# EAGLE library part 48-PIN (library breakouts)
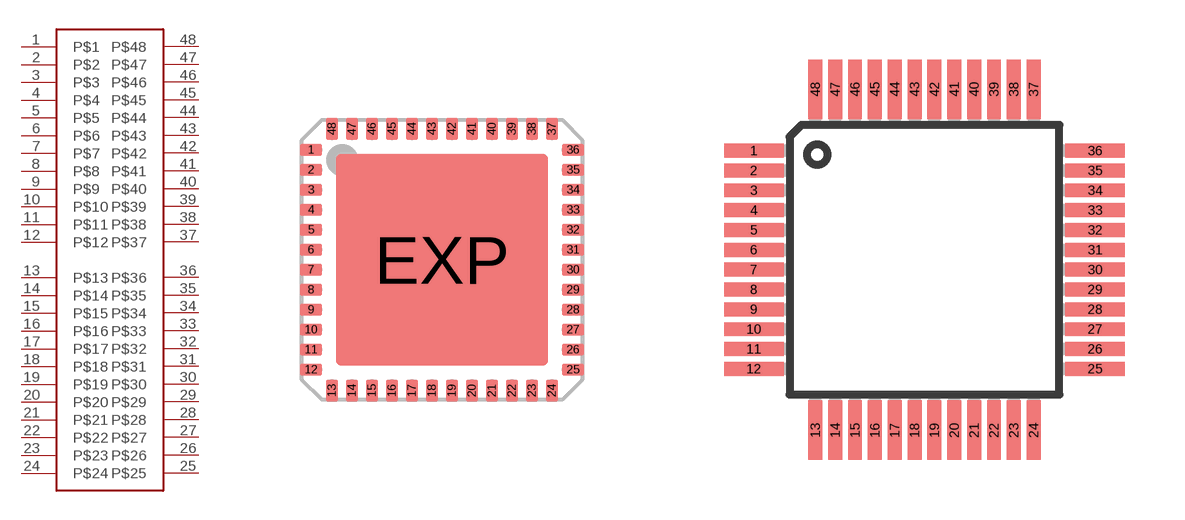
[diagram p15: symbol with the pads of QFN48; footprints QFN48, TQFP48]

Designator prefix -

## 48-PINQFN  [QFN48]
1  P$1
2  P$2
3  P$3
4  P$4
5  P$5
6  P$6
7  P$7
8  P$8
9  P$9
10  P$10
11  P$11
12  P$12
13  P$13
14  P$14
15  P$15
16  P$16
17  P$17
18  P$18
19  P$19
20  P$20
21  P$21
22  P$22
23  P$23
24  P$24
25  P$25
26  P$26
27  P$27
28  P$28
29  P$29
30  P$30
31  P$31
32  P$32
33  P$33
34  P$34
35  P$35
36  P$36
37  P$37
38  P$38
39  P$39
40  P$40
41  P$41
42  P$42
43  P$43
44  P$44
45  P$45
46  P$46
47  P$47
48  P$48

## 48-PINTQFP  [TQFP48]
Pads as for QFN48

## Footprint QFN48 (pad centres in mm)
48-pin QFN 7 x 7 mm LF48 48 Quad Flat Package No Leads Source: http://v4.cypress.com/cfuploads/img/products/cywusb6934.pdf
smd 0.55 x 0.3: 1 -3.275,2.75; 2 -3.275,2.25; 3 -3.275,1.75; 4 -3.275,1.25; 5 -3.275,0.75; 6 -3.275,0.25; 7 -3.275,-0.25; 8 -3.275,-0.75; 9 -3.275,-1.25; 10 -3.275,-1.75; 11 -3.275,-2.25; 12 -3.275,-2.75; 25 3.275,-2.75; 26 3.275,-2.25; 27 3.275,-1.75; 28 3.275,-1.25; 29 3.275,-0.75; 30 3.275,-0.25; 31 3.275,0.25; 32 3.275,0.75; 33 3.275,1.25; 34 3.275,1.75; 35 3.275,2.25; 36 3.275,2.75
smd 0.3 x 0.55: 13 -2.75,-3.275; 14 -2.25,-3.275; 15 -1.75,-3.275; 16 -1.25,-3.275; 17 -0.75,-3.275; 18 -0.25,-3.275; 19 0.25,-3.275; 20 0.75,-3.275; 21 1.25,-3.275; 22 1.75,-3.275; 23 2.25,-3.275; 24 2.75,-3.275; 37 2.75,3.275; 38 2.25,3.275; 39 1.75,3.275; 40 1.25,3.275; 41 0.75,3.275; 42 0.25,3.275; 43 -0.25,3.275; 44 -0.75,3.275; 45 -1.25,3.275; 46 -1.75,3.275; 47 -2.25,3.275; 48 -2.75,3.275
smd 5.309 x 5.309: EXP 0,0

## Footprint TQFP48 (pad centres in mm)
THIN QUAD FLAT PACK
smd 1.5 x 0.35: 1 -4.3,2.75; 2 -4.3,2.25; 3 -4.3,1.75; 4 -4.3,1.25; 5 -4.3,0.75; 6 -4.3,0.25; 7 -4.3,-0.25; 8 -4.3,-0.75; 9 -4.3,-1.25; 10 -4.3,-1.75; 11 -4.3,-2.25; 12 -4.3,-2.75; 25 4.3,-2.75; 26 4.3,-2.25; 27 4.3,-1.75; 28 4.3,-1.25; 29 4.3,-0.75; 30 4.3,-0.25; 31 4.3,0.25; 32 4.3,0.75; 33 4.3,1.25; 34 4.3,1.75; 35 4.3,2.25; 36 4.3,2.75
smd 0.35 x 1.5: 13 -2.75,-4.3; 14 -2.25,-4.3; 15 -1.75,-4.3; 16 -1.25,-4.3; 17 -0.75,-4.3; 18 -0.25,-4.3; 19 0.25,-4.3; 20 0.75,-4.3; 21 1.25,-4.3; 22 1.75,-4.3; 23 2.25,-4.3; 24 2.75,-4.3; 37 2.75,4.3; 38 2.25,4.3; 39 1.75,4.3; 40 1.25,4.3; 41 0.75,4.3; 42 0.25,4.3; 43 -0.25,4.3; 44 -0.75,4.3; 45 -1.25,4.3; 46 -1.75,4.3; 47 -2.25,4.3; 48 -2.75,4.3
